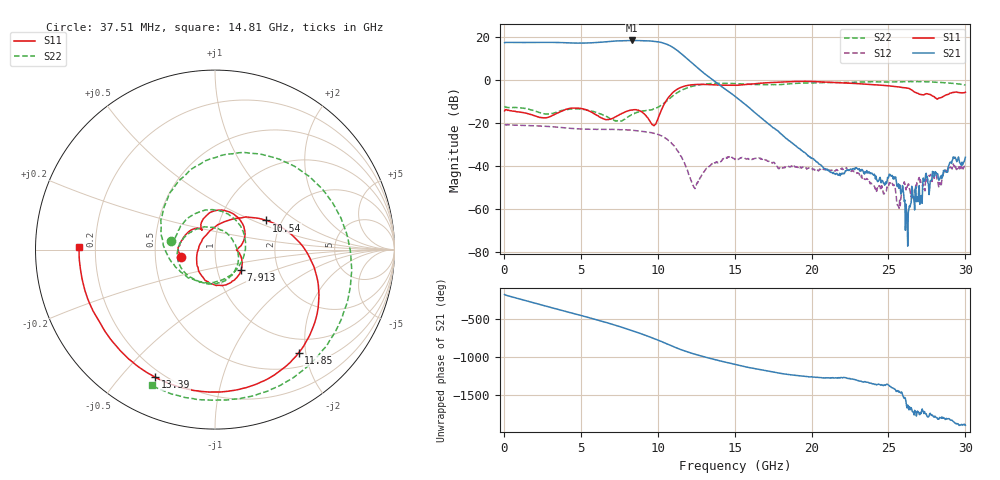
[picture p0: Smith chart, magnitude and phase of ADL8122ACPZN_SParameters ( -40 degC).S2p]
! "Analog Devices, Inc."
! Device:	ADL8122ACPZN
! Description:	"10 kHz to 10 GHz, Wideband, Low Noise Amplifier"
! Conditions:	Vdd = 5.0 V
!		IDQ = 95 mA
!		Pin = -25 dBm
!		Operating Temperature = +25 C (at package bottom)
! Product validation unit SN1 soldered down to Evaluation Board as shown on ADL8122-EVALZ User Guide. Board loss de-embedded from S21 magnitude.  All other RF measurements reference to RF coaxial connector.
! Frequency (GHz)	S11_Mag (dB)	S11_Phase (deg)	S21_Mag (dB)	S21_Phase (deg)	S12_Mag (dB)	S12_Phase (deg)	S22_Mag (dB)	S22_Phase (deg)
#  GHZ  S  DB  R 50
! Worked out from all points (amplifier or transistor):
!   800 points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, 37.51 MHz to 30 GHz, reference 50 ohm
!   highest |S21| = 18.4 dB at 8.325 GHz (marker M1)
!   |S21| within 3 dB of that: start of sweep to 10.93 GHz
!   unconditionally stable (mu >= 1): start of sweep to end of sweep
!   at 5.025 GHz: K = 1.17, MAG = 17.5 dB, |S12| = -22.8 dB
!   at 15.04 GHz: K = 10.23, MAG = 1.4 dB, |S12| = -36.6 dB
!   at 30 GHz: K = 780.10, MAG = -30.5 dB, |S12| = -38.7 dB
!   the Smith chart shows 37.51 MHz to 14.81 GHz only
!   S11 on the Smith chart (normalised r, x): 37.51 MHz: 0.68, -0.06; 7.913 GHz: 1.30, -0.31; 10.54 GHz: 1.66, +0.60; 11.85 GHz: 0.74, -1.87; 13.39 GHz: 0.17, -0.62; 14.81 GHz: 0.14, +0.01
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0.03750899  -14.30 -167.1  17.39 -177.5  -20.86 2.9  -12.10 169.2
1.575009  -15.69 135.4  17.47 93.6  -21.16 -75.1  -13.49 71.7
2.250008  -17.13 124.4  17.50 56.6  -21.32 -107.5  -14.98 20.7
3.075008  -16.75 122.4  17.52 11.0  -21.67 -148.4  -15.58 -57.1
4.162508  -13.35 91.1  17.31 -48.0  -22.33 157.9  -13.65 -136.7
5.062508  -13.30 50.5  17.17 -95.6  -22.73 114.1  -13.53 -174.9
5.812507  -15.40 18.3  17.38 -136.6  -22.91 75.9  -14.55 159.9
6.637507  -18.44 0.1  17.79 176.1  -22.92 33.0  -16.84 121.2
7.237507  -17.09 -9.6  18.14 139.5  -22.93 -0.2  -18.81 68.8
7.912507  -14.66 -37.8  18.37 95.7  -23.13 -38.6  -17.88 -6.0
8.325006  -13.99 -61.1  18.41 68.2  -23.32 -62.8  -16.13 -42.2
9.225006  -16.49 -127.4  18.28 4.8  -24.05 -116.7  -14.16 -102.2
10.05001  -17.11 83.7  17.74 -59.3  -25.39 -173.6  -12.40 -155.7
10.53751  -9.69 29.7  16.77 -100.8  -27.24 149.5  -9.98 161.8
11.10001  -5.04 -9.8  14.63 -149.1  -30.99 103.4  -6.65 107.2
11.85001  -2.62 -51.0  10.27 153.9  -40.64 40.9  -3.76 43.1
13.3875  -2.10 -115.2  1.06 64.5  -39.82 -177.1  -1.65 -49.4
14.8125  -2.41 178.7  -6.42 -6.0  -35.91 105.0  -1.58 -114.8
15.0375  -2.40 167.4  -7.63 -16.8  -36.60 96.5  -1.62 -124.4
20.025  -0.65 16.7  -36.48 -178.1  -40.90 -62.4  -1.35 47.2
25.0125  -2.68 -114.7  -45.08 71.7  -49.08 148.9  -0.89 -104.7
30  -5.64 -96.6  -35.87 -95.0  -38.69 -93.4  -2.23 -163.2
